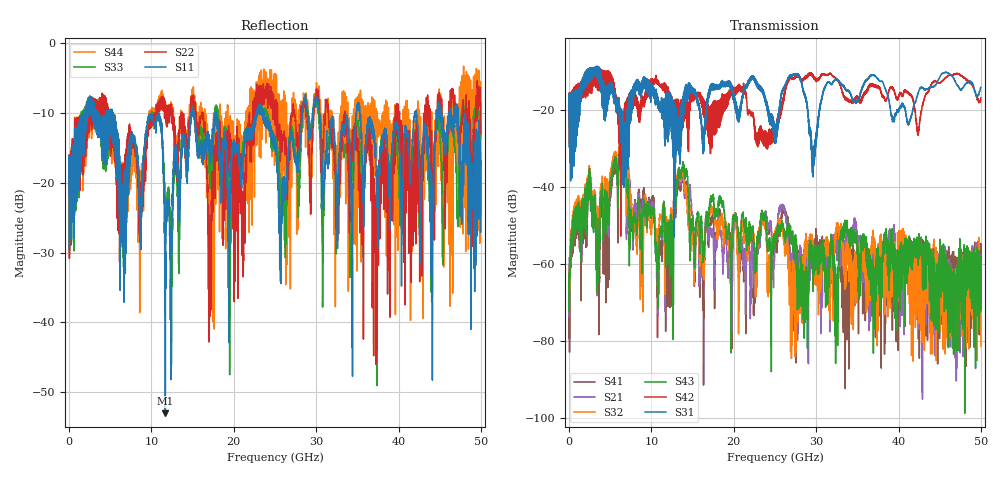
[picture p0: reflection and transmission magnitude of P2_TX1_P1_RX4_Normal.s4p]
!Keysight Technologies,N5225B,MY57041031,A.13.20.10
!Date: Friday, May 31, 2019 11:19:42
!Correction: S11(Full 4 Port(1,2,3,4))
!S12(Full 4 Port(1,2,3,4))
!S13(Full 4 Port(1,2,3,4))
!S14(Full 4 Port(1,2,3,4))
!S21(Full 4 Port(1,2,3,4))
!S22(Full 4 Port(1,2,3,4))
!S23(Full 4 Port(1,2,3,4))
!S24(Full 4 Port(1,2,3,4))
!S31(Full 4 Port(1,2,3,4))
!S32(Full 4 Port(1,2,3,4))
!S33(Full 4 Port(1,2,3,4))
!S34(Full 4 Port(1,2,3,4))
!S41(Full 4 Port(1,2,3,4))
!S42(Full 4 Port(1,2,3,4))
!S43(Full 4 Port(1,2,3,4))
!S44(Full 4 Port(1,2,3,4))
!S4P File: Measurements: <S11,S12,S13,S14>,
!<S21,S22,S23,S24>,
!<S31,S32,S33,S34>,
!<S41,S42,S43,S44>:
# Hz S  dB  R 50.0
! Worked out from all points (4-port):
!   5000 points, 10 MHz to 50 GHz, reference 50 ohm
!   strongest paths, dB at 10 MHz, 12.51 GHz, 25.01 GHz, 37.51 GHz, 50 GHz:
!     S31: -19.5, -17.3, -28.8, -12.1, -14.3
!     S42: -19.5, -19.1, -25.3, -14.3, -16.9
!     S43: -64.7, -48.8, -56.0, -59.5, -60.1
!     S32: -61.7, -47.2, -53.4, -54.9, -81.4
!     S21: -58.4, -48.7, -54.4, -58.1, -67.3
!     S41: -67.9, -53.3, -54.6, -58.3, -58.6
!   lowest |S11| = -53.0 dB at 11.69 GHz (marker M1), VSWR 1.00, Z = 49.8 - j0.111 ohm
!   |S11| at or under -10 dB: 5.36 GHz to 10.81 GHz (5.449 GHz wide, 67.4 % of centre); 17.89 GHz to 22.7 GHz (4.805 GHz wide, 23.7 % of centre); 35.31 GHz to 41.96 GHz (6.644 GHz wide, 17.2 % of centre)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
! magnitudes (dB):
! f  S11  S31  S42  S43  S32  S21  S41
! 10 MHz  -19.6  -19.5  -19.5  -64.7  -61.7  -58.4  -67.9
! 6.27 GHz  -23.1  -20.3  -52.9  -29.8  -28.5  -29.7  -30.9
! 8.81 GHz  -22.3  -12.9  -19.7  -51.2  -54.3  -51.4  -46.5
! 11.69 GHz  -53.0  -22.9  -15.2  -52.7  -54.0  -55.6  -58.6
! 17.06 GHz  -15.3  -15.9  -21.2  -44.6  -46.7  -50.4  -49.7
! 23.05 GHz  -8.7  -14.5  -28.7  -54.3  -52.1  -54.4  -55.7
! 50 GHz  -17.2  -14.3  -16.9  -60.1  -81.4  -67.3  -58.6
